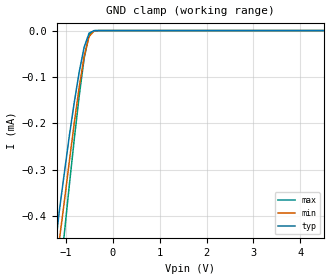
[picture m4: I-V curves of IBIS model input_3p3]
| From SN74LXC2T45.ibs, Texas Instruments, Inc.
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|   input_3p3 Model
[Model]   input_3p3
Model_type   Input
Vinl = 1.5
Vinh = 2.1
|   typ   min   max
C_comp   2.94pF   2.39pF   3.86pF
| Where Nom  PVT is Nominal Process, 3.3V, 27C
|   Fast PVT is Strong Process,  3.6V, -55C
|   Slow PVT is Weak Process,   3.0V, 150C
[Voltage Range]   3.3   2.97   3.63
|Junction Temperature
[Temperature Range]   25   125   -40
[GND Clamp Reference]   0   0   0
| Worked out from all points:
|   GND clamp passes 1 mA (typ) near -1.81 V on its own axis
[GND Clamp]
|   Voltage   I(typ)   I(min)   I(max)
-2.5V     -1.66mA    -1.64mA    -2.09mA
-1.24V    -478uA     -541uA     -650uA
-1.14V    -389uA     -453uA     -542uA
-1.03V    -305uA     -366uA     -435uA
-925mV    -226uA     -281uA     -332uA
-820mV    -154uA     -198uA     -233uA
-715mV    -88.7uA    -121uA     -140uA
-610mV    -35.6uA    -54.9uA    -59.7uA
-505mV    -5.5uA     -12.7uA    -8.49uA
-400mV    -210nA     -1.14uA    -141nA
8V        3.61nA     3.43nA     4.22nA
